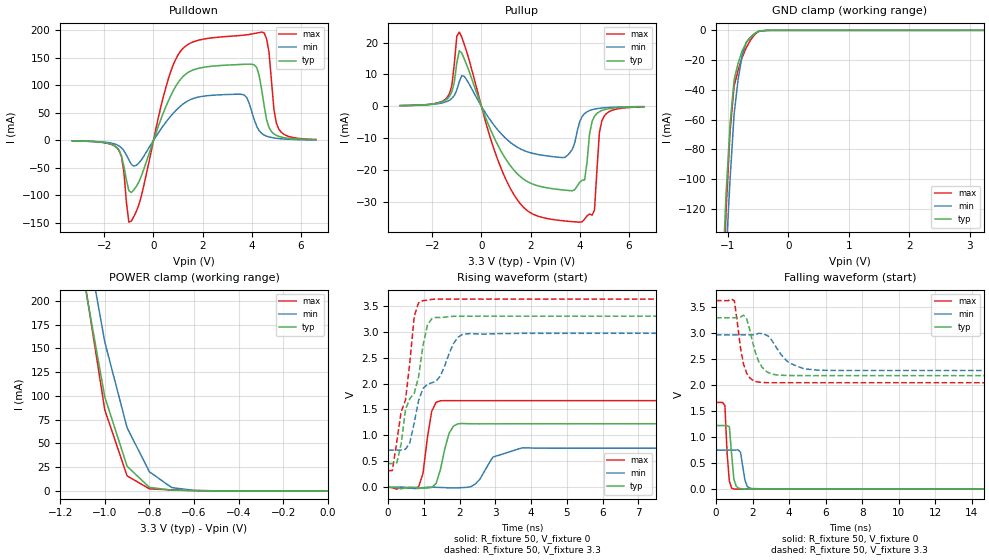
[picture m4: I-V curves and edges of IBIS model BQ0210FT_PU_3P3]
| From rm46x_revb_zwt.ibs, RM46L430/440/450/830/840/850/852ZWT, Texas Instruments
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|   Model Cell BQ0210FT_PU_3P3
|BQ0210FT_PU_3P3
[Model]   BQ0210FT_PU_3P3
Model_type   I/O
Polarity   Non-Inverting
Enable   Active-Low
Vinl =  1.15
Vinh =  1.55
Cref =  15.0001pF
Rref =  101.0000M
Vref =  0V
Vmeas =  1.65
C_comp   1.2p   1.2p   1.2p
[Model Spec]
Vinl   1.15   1.02   1.28
Vinh   1.55   1.45   1.65
[Temperature Range]   25   155   -40
[Voltage Range]   3.3   2.97   3.63
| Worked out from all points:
|   slope of the pulldown table from 0 to 0.495 V, typ, clamps not added: 8.21 ohm
|   slope of the pullup table from 0 to 0.495 V, typ, clamps not added: 52.1 ohm
|   GND clamp passes 1 mA (typ) near -0.51 V on its own axis
|   POWER clamp passes 1 mA (typ) near -0.71 V on its own axis
|   rising waveform, R_fixture 50, V_fixture 0: 20-80 % time 262ps typ, 466ps min, 201ps max; typ from 0 V to 1.23 V
|   rising waveform, R_fixture 50, V_fixture 3.3: 20-80 % time 576ps typ, 968ps min, 420ps max; typ from 0.458 V to 3.3 V
|   falling waveform, R_fixture 50, V_fixture 0: 20-80 % time 181ps typ, 214ps min, 167ps max; typ from 1.23 V to 0 V
|   falling waveform, R_fixture 50, V_fixture 3.3: 20-80 % time 29.5ns typ, 31.8ns min, 18.4ns max; typ from 3.3 V to 0.466 V
[POWER_clamp]
|   voltage   I(typ)   I(min)   I(max)
-3.3V     4.048A     4.625A     4.878A
-1.1V     231mA      288.4mA    235.6mA
-1.067V   187mA      244.6mA    185.5mA
-1.033V   143mA      200.7mA    135.4mA
-1V       98.97mA    156.8mA    85.31mA
-900mV    25.98mA    66.53mA    15.85mA
-800mV    3.682mA    20.17mA    2.197mA
-700mV    854.4uA    3.509mA    1.047mA
-600mV    293.2uA    571.4uA    381uA
0V        544.7pA    9.476nA    486.3pA
[Pulldown]
|   voltage   I(typ)   I(min)   I(max)
-3.3V     -969uA     -848.2uA   -928.8uA
-1.4V     -17.91mA   -9.953mA   -18.22mA
-1V       -91.46mA   -35.59mA   -148.6mA
-900mV    -94.7mA    -43.39mA   -146.6mA
1.1V      110.9mA    62.3mA     162mA
3.7V      138.3mA    82.11mA    191.3mA
4.2V      132.3mA    25.59mA    195mA
4.4V      92.36mA    12.74mA    196.7mA
4.7V      23.23mA    6.307mA    159.7mA
4.9V      11.73mA    4.459mA    55.98mA
5.1V      7.323mA    3.326mA    20.29mA
6.6V      1.15mA     841.4uA    1.761mA
[Pullup]
|   voltage   I(typ)   I(min)   I(max)
-3.3V     170.4uA    161.9uA    202.8uA
-1.4V     2.221mA    1.492mA    2.652mA
-900mV    17.47mA    7.707mA    23.31mA
500mV     -9.587mA   -5.844mA   -13.22mA
1.4V      -20.78mA   -12.62mA   -28.76mA
3.4V      -26.42mA   -16.07mA   -36.11mA
4V        -23.95mA   -4.814mA   -36.5mA
4.2V      -23.22mA   -2.294mA   -35.5mA
4.6V      -3.167mA   -930.7uA   -32.71mA
4.8V      -1.739mA   -669.4uA   -8.284mA
5V        -1.12mA    -503.2uA   -3.036mA
6.6V      -167.4uA   -126.3uA   -220.9uA
[GND_clamp]
|   voltage   I(typ)   I(min)   I(max)
-3.3V     -3.252A    -2.876A    -4.947A
-1.1V     -174mA     -209.6mA   -199.1mA
-1.033V   -110.1mA   -151.3mA   -121.8mA
-966.7mV  -63.24mA   -100.2mA   -67.92mA
-900mV    -33.37mA   -56.39mA   -37.45mA
-833.3mV  -22.09mA   -33.02mA   -26.82mA
-766.7mV  -13.8mA    -16.89mA   -18.25mA
-700mV    -8.501mA   -8.011mA   -11.77mA
-566.7mV  -2.409mA   -2.408mA   -3.203mA
-500mV    -646.1uA   -915.3uA   -753.3uA
-300mV    -20.81uA   -21.61uA   -33.46uA
3.233V    -1.13uA    4.04uA     -9.303uA
[Ramp]
| variable   typ   min   max
dV/dt_f   1.74033/29.50484n   0.5633648/0.4686342n   2.03012/18.34879n
dV/dt_r   0.757745/0.2542626n  0.4747336/0.4320037n   1.026673/0.1940422n
R_load = 50
[Rising Waveform]
R_fixture = 50
V_fixture = 0
V_fixture_min = 0
V_fixture_max = 0
|   time   V(typ)   V(min)   V(max)
0s        106.2uV    102.3uV    130.5uV
852ps     -8.99mV    -23.3mV    5.233mV
976ps     -18.17mV   -6.949mV   263.7mV
1.22ns    -3.038mV   1.271mV    1.465V
1.464ns   341.6mV    -3.793mV   1.668V
1.708ns   1.043V     -11.13mV   1.671V
2.076ns   1.23V      -6.999mV   1.67V
2.932ns   1.224V     581.8mV    1.67V
3.744ns   1.225V     759.3mV    1.67V
35.6ns    1.225V     753.7mV    1.671V
[Rising Waveform]
R_fixture = 50
V_fixture = 3.3
V_fixture_min = 2.97
V_fixture_max = 3.63
|   time   V(typ)   V(min)   V(max)
0s        457.7mV    717.2mV    322.1mV
120ps     457.7mV    717.2mV    321.5mV
244ps     469.8mV    717.2mV    878.1mV
488ps     1.506V     734.4mV    1.683V
732ps     1.814V     1.243V     3.296V
976ps     2.73V      1.904V     3.601V
1.22ns    3.251V     2.014V     3.624V
1.956ns   3.299V     2.894V     3.63V
2.32ns    3.299V     2.964V     3.63V
35.6ns    3.3V       2.97V      3.63V
[Falling Waveform]
R_fixture = 50
V_fixture = 0
V_fixture_min = 0
V_fixture_max = 0
|   time   V(typ)   V(min)   V(max)
0s        1.225V     753.6mV    1.671V
488ps     1.225V     753.6mV    1.609V
608ps     1.224V     753.6mV    695.8mV
732ps     1.202V     753.6mV    154.3mV
976ps     200.8mV    752.9mV    3.766mV
1.1ns     62.07mV    753.3mV    1.669mV
1.344ns   9.506mV    706.8mV    1.259mV
1.588ns   2.551mV    165.6mV    1.419mV
1.956ns   1.086mV    12.77mV    1.097mV
35.6ns    284.8uV    261.3uV    136.6uV
[Falling Waveform]
R_fixture = 50
V_fixture = 3.3
V_fixture_min = 2.97
V_fixture_max = 3.63
|   time   V(typ)   V(min)   V(max)
0s        3.3V       2.97V      3.63V
1.008ns   3.299V     2.97V      3.628V
1.512ns   3.35V      2.97V      2.402V
2.18ns    2.606V     2.977V     2.073V
18.06ns   2.186V     2.285V     2.052V
20.81ns   2.186V     2.285V     477.5mV
29.14ns   2.189V     2.285V     345.2mV
34.82ns   551.6mV    2.285V     345mV
35.92ns   525.6mV    755.6mV    345mV
36.8ns    465.6mV    755.6mV    345mV
